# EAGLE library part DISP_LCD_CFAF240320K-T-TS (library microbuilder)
Footprint courtesy Morten Hjerde
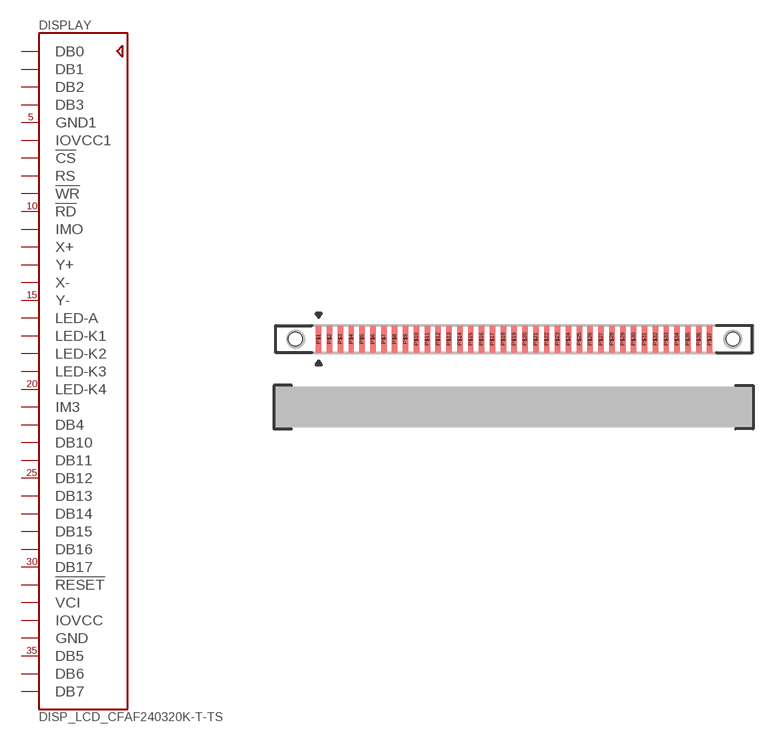
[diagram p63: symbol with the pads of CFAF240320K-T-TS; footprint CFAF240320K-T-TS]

Designator prefix DISPLAY

## DISP_LCD_CFAF240320K-T-TS  [CFAF240320K-T-TS]
P$1  DB0  pas
P$2  DB1  pas
P$3  DB2  pas
P$4  DB3  pas
P$5  GND1  pwr
P$6  IOVCC1  pwr
P$7  !CS  pas
P$8  RS  pas
P$9  !WR  pas
P$10  !RD  pas
P$11  IMO  pas
P$12  X+  pas
P$13  Y+  pas
P$14  X-  pas
P$15  Y-  pas
P$16  LED-A  pas
P$17  LED-K1  pas
P$18  LED-K2  pas
P$19  LED-K3  pas
P$20  LED-K4  pas
P$21  IM3  pas
P$22  DB4  pas
P$23  DB10  pas
P$24  DB11  pas
P$25  DB12  pas
P$26  DB13  pas
P$27  DB14  pas
P$28  DB15  pas
P$29  DB16  pas
P$30  DB17  pas
P$31  !RESET  pas
P$32  VCI  pwr
P$33  IOVCC  pwr
P$34  GND  pwr
P$35  DB5  pas
P$36  DB6  pas
P$37  DB7  pas

## Footprint CFAF240320K-T-TS (pad centres in mm)
smd 0.4 x 2: P$1 0,0; P$2 0.8,0; P$3 1.6,0; P$4 2.4,0; P$5 3.2,0; P$6 4,0; P$7 4.8,0; P$8 5.6,0; P$9 6.4,0; P$10 7.2,0; P$11 8,0; P$12 8.8,0; P$13 9.6,0; P$14 10.4,0; P$15 11.2,0; P$16 12,0; P$17 12.8,0; P$18 13.6,0; P$19 14.4,0; P$20 15.2,0; P$21 16,0; P$22 16.8,0; P$23 17.6,0; P$24 18.4,0; P$25 19.2,0; P$26 20,0; P$27 20.8,0; P$28 21.6,0; P$29 22.4,0; P$30 23.2,0; P$31 24,0; P$32 24.8,0; P$33 25.6,0; P$34 26.4,0; P$35 27.2,0; P$36 28,0; P$37 28.8,0
hole 1 at -1.725,0
hole 1 at 30.53,0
